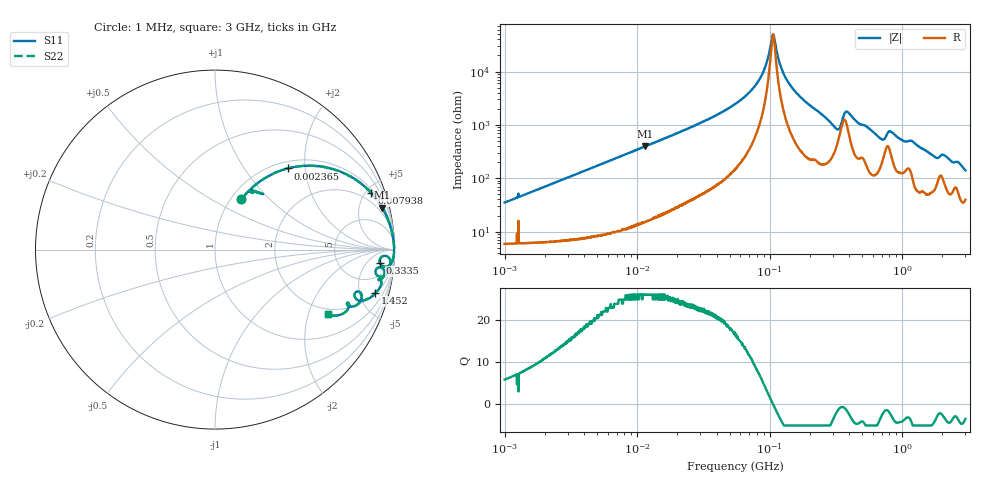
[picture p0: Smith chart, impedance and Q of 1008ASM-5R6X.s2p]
!s-Parameter Generated by FASTRON Sdn. Bhd.
!FASTRON P/N : 1008ASM-5R6X
!Keysight Technologies: E4991B_MY54100416_A.01.15
!Date: Wed Jun 19 15:37:19 2024
!Version  :Rev00  Wed Jun 19 15:37:19 2024
!Data & Calibration Information:
!Freq  S11  S21  S12  S22
!PortZ  Port1:50+j0  Port2:50+j0
!When reading reference impedance value at option line is always used.
! Remarks : This data is being provided solely for informational purposes.
# Hz S dB R 50
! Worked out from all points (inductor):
!   1601 points, 1 MHz to 3 GHz, reference 50 ohm
!   read as one part in series: L = 5.49 uH near 1.041 MHz
!   highest Q = 26 at 11.5 MHz (marker M1), where L = 5.48 uH
!   self-resonance near 106 MHz
!   S11 on the Smith chart (normalised r, x): 1 MHz: 1.12, +0.69; 2.365 MHz: 1.13, +1.63; 7.938 MHz: 1.22, +5.44; 333.5 MHz: 13, -12; 1.452 GHz: 2.12, -6.91; 3 GHz: 1.79, -2.71
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1000000  -10.00 62.2  -0.94 -18.1  -0.94 -18.1  -10.00 62.2
2364779  -4.31 48.0  -2.55 -37.4  -2.55 -37.4  -4.31 48.0
3804036  -2.23 36.2  -4.56 -50.6  -4.56 -50.6  -2.23 36.2
7937891  -0.66 19.9  -9.36 -67.8  -9.36 -67.8  -0.66 19.9
1.149534e7  -0.35 14.1  -12.30 -73.7  -12.30 -73.7  -0.35 14.1
1.447069e7  -0.24 11.2  -14.20 -76.5  -14.20 -76.5  -0.24 11.2
5.504702e7  -0.03 2.3  -27.90 -84.2  -27.90 -84.2  -0.03 2.3
8.380746e7  -0.02 0.8  -37.10 -81.1  -37.10 -81.1  -0.02 0.8
9.309362e7  -0.02 0.4  -42.00 -75.1  -42.00 -75.1  -0.02 0.4
1.060286e8  -0.02 0.0  -53.90 -3.5  -53.90 -3.5  -0.02 0.0
1.092603e8  -0.02 -0.1  -51.60 38.4  -51.60 38.4  -0.02 -0.1
1.213667e8  -0.02 -0.4  -41.80 74.4  -41.80 74.4  -0.02 -0.4
1.341416e8  -0.02 -0.8  -37.10 79.9  -37.10 79.9  -0.02 -0.8
2.083556e8  -0.05 -2.6  -26.80 81.5  -26.80 81.5  -0.05 -2.6
3.334925e8  -0.71 -4.6  -19.20 42.0  -19.20 42.0  -0.71 -4.6
3.817355e8  -0.28 -2.6  -25.30 52.8  -25.30 52.8  -0.28 -2.6
6.855309e8  -0.56 -9.3  -15.50 63.8  -15.50 63.8  -0.56 -9.3
7.925923e8  -0.62 -6.1  -18.10 53.5  -18.10 53.5  -0.62 -6.1
1.452135e9  -0.69 -15.1  -11.50 65.8  -11.50 65.8  -0.69 -15.1
1.782824e9  -1.39 -19.5  -9.24 55.3  -9.24 55.3  -1.39 -19.5
2.050964e9  -1.36 -17.1  -10.10 54.0  -10.10 54.0  -1.36 -17.1
3e9  -2.79 -29.6  -5.76 44.1  -5.76 44.1  -2.79 -29.6
